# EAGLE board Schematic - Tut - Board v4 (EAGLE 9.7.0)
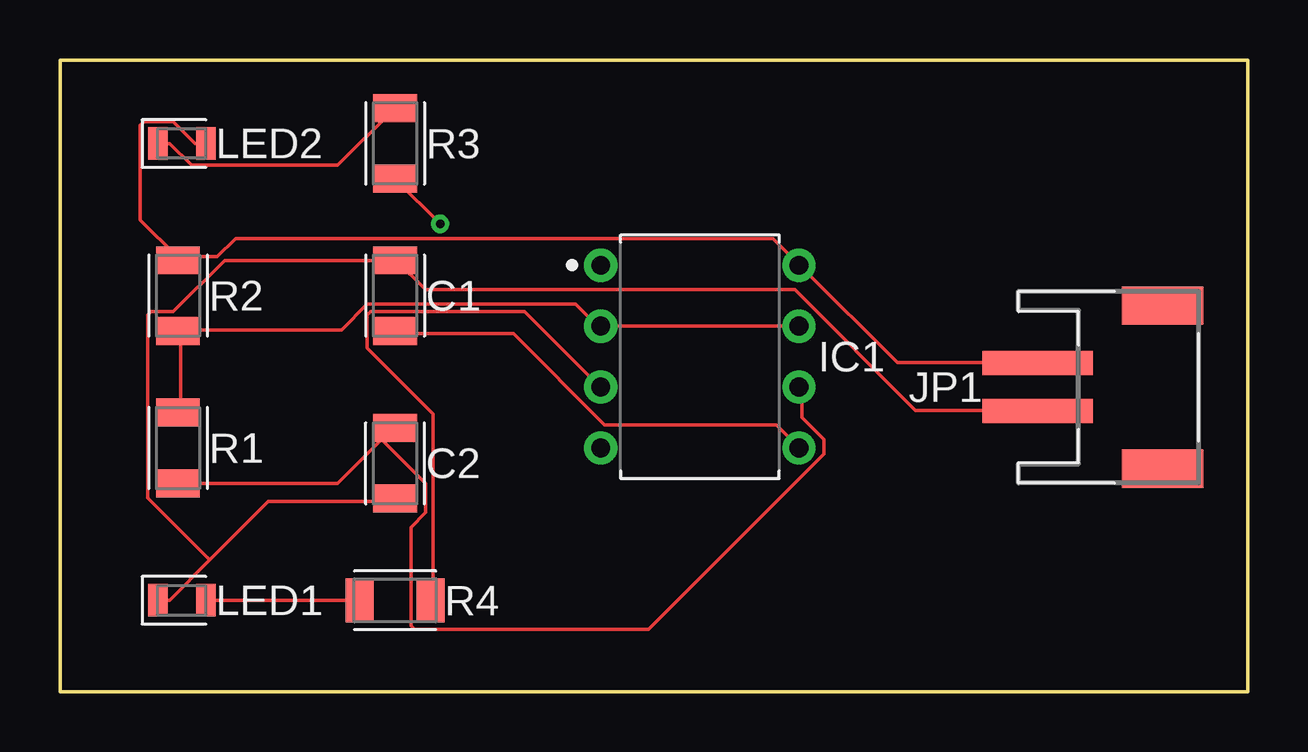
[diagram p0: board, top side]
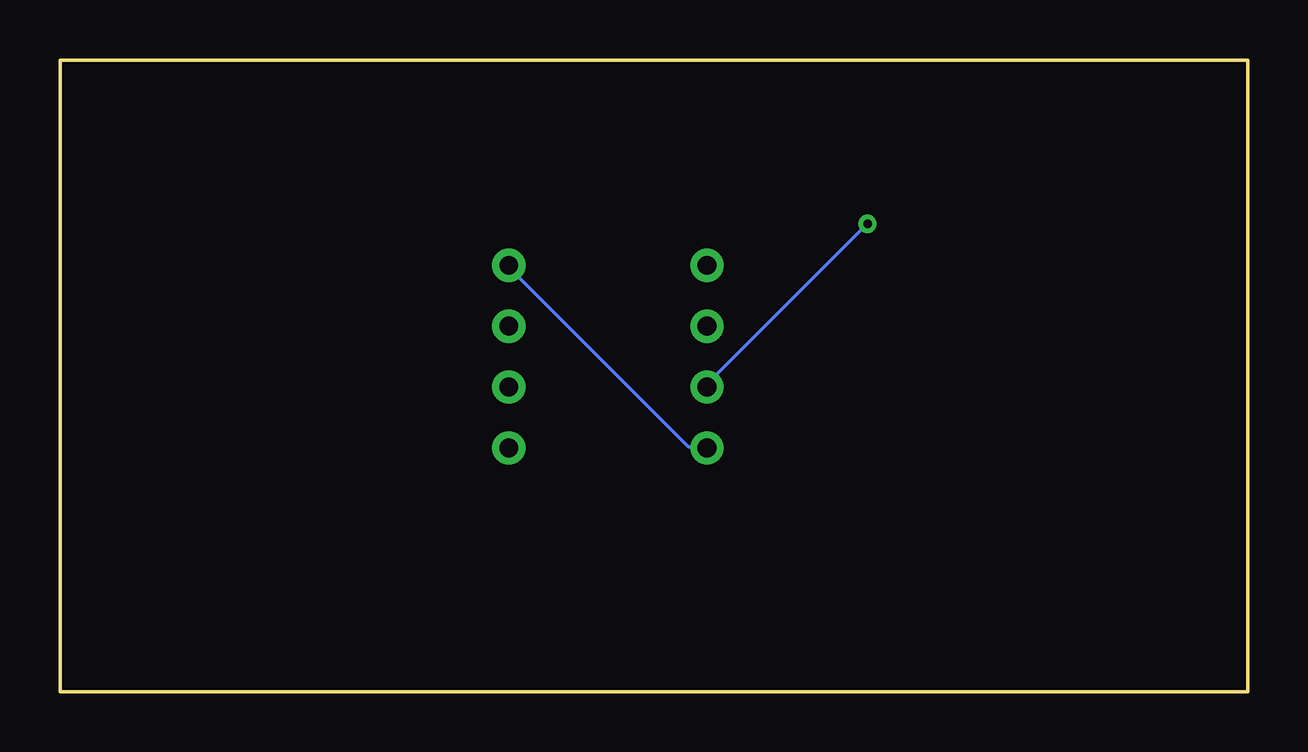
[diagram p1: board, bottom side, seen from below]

Size 49.51 x 26.34 mm. Coordinates in mm from the lower left corner, seen from the top.
Outline: 49.51,0 49.51,26.34 0,26.34 0,0 49.51,0
Copper layers (1*16): Top 0.035mm / dielectric 1.5mm / Bottom 0.035mm
Design rules "Fusion Electronics Design Rules": minimum track width 6mil, minimum drill 0.35mm, track to track 6mil, track to pad 6mil, pad to pad 6mil, via to via 6mil, smd to smd 6mil, copper to edge 40mil, drill to drill 6mil, minimum pad ring 10mil, minimum via ring 8mil, stop-mask expansion 4mil, vias tented up to drill 0mil, thermal gap 10mil

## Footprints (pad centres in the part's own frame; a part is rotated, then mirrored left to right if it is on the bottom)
CAPC3216X135 = smd 1.165 x 1.815: 1 -1.475,0; 2 1.475,0
P(R-PDIP-T8) = drill 0.786 pad 1.386: 1 -4.13,3.81; 2 -4.13,1.27; 3 -4.13,-1.27; 4 -4.13,-3.81; 5 4.13,-3.81; 6 4.13,-1.27; 7 4.13,1.27; 8 4.13,3.81
JSTPH2 = smd 1 x 4.6: 1 -1,-3.7; 2 1,-3.7 | smd 1.6 x 3.4: NC1 -3.4,1.5; NC2 3.4,1.5
LEDC2012X110N_B = smd 0.817 x 1.352: 1 -1,0 | smd 0.822 x 1.352: 2 0.998,0
RESC3216X70 = smd 1.165 x 1.815: 1 -1.475,0; 2 1.475,0

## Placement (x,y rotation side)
C1  10n  [CAPC3216X135]  13.97,16.51 90 top
C2  1u  [CAPC3216X135]  13.97,9.53 270 top
IC1  IC-555  [P(R-PDIP-T8)]  26.67,13.97 0 top
JP1  JST-PH2  [JSTPH2]  44.45,12.7 270 top
LED1  LED-BLUE  [LEDC2012X110N_B]  5.08,3.81 0 top
LED2  LED-BLUE  [LEDC2012X110N_B]  5.08,22.86 0 top
R1  470k  [RESC3216X70]  4.92,10.16 90 top
R2  1k  [RESC3216X70]  4.92,16.51 90 top
R3  220  [RESC3216X70]  13.97,22.86 90 top
R4  220  [RESC3216X70]  13.97,3.81 0 top

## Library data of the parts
C1 C2 = Tutorial - Fusion 360; CATEGORY: Capacitor
IC1 JP1 = Tutorial - Fusion 360
LED1 LED2 = Tutorial - Fusion 360; CATEGORY: Opto-Electronic; COLOR: Blue; SUB-CATEGORY: LED
R1-R4 = Tutorial - Fusion 360; CATEGORY: Resistor; SUB-CATEGORY: Fixed

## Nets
GND: C1.2 C2.2 JP1.2 LED1.1
N$1: C1.1 IC1.5
N$2: IC1.2 IC1.7 R1.2 R2.1
N$3: C2.1 IC1.6 R1.1
N$4: IC1.3 R3.1 R4.2
N$5: LED2.1 R3.2
N$6: LED1.2 R4.1
N$8: IC1.1
VSS: IC1.4 IC1.8 JP1.1 LED2.2 R2.2

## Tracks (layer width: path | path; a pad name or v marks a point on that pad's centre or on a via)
GND
  Top 0.152: LED1.1 4.57,3.81 6.25,5.49 | 6.25,5.49 8.69,7.92 13.87,7.92 C2.2 | 6.25,5.49 3.66,8.08 3.66,15.7 3.81,15.85 4.72,15.85 6.86,17.98 13.87,17.98 C1.2 14.02,17.98 15.24,16.76 30.63,16.76 35.66,11.73 40.69,11.73 JP1.2
N$1
  Top 0.152: C1.1 14.02,14.94 18.9,14.94 22.71,11.12 29.87,11.12 30.79,10.21 IC1.5
N$2
  Top 0.152: R1.2 5.03,11.73 5.03,14.94 R2.1 5.03,15.09 11.73,15.09 12.8,16.15 21.49,16.15 22.4,15.24 IC1.2 IC1.7
N$3
  Top 0.152: 13.41,10.52 13.87,10.97 C2.1 13.41,10.52 | 13.41,10.52 11.58,8.69 5.03,8.69 R1.1 | 13.41,10.52 15.24,8.69 15.24,7.47 14.63,6.86 14.63,2.74 14.78,2.59 24.54,2.59 31.85,9.91 31.85,10.52 30.94,11.43 30.94,12.65 IC1.6
N$4  (via drill 0.35)
  Top 0.152: v15.85,19.51 14.02,21.34 R3.1 | R4.2 15.54,3.81 15.54,11.58 12.8,14.33 12.8,15.7 12.95,15.85 19.36,15.85 22.4,12.8 IC1.3
  Bottom 0.152: v15.85,19.51 22.55,12.8 IC1.3
N$5
  Top 0.152: LED2.1 4.57,22.86 5.49,21.95 11.58,21.95 13.87,24.23 R3.2
N$6
  Top 0.152: R4.1 LED1.2
VSS
  Top 0.152: LED2.2 5.64,22.86 4.72,23.77 3.5,23.77 3.35,23.62 3.35,19.66 4.88,18.14 R2.2 5.03,18.14 6.55,18.14 7.32,18.9 29.72,18.9 30.79,17.83 IC1.8 30.94,17.68 34.9,13.72 40.69,13.72 JP1.1
  Bottom 0.152: IC1.4 22.55,10.21 23.32,10.21 30.79,17.68 IC1.8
